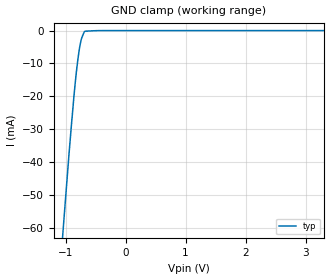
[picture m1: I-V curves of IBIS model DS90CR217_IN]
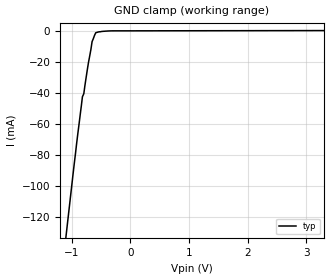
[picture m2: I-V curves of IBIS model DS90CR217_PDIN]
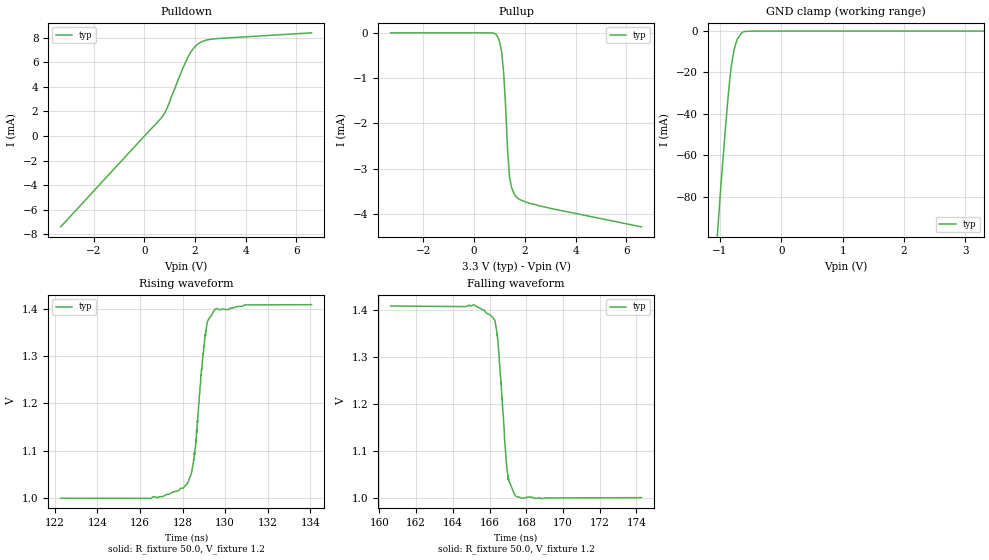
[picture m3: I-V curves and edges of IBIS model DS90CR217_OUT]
|   National Semiconductor Corporation
|   Interface Products Group
|   IBIS Model of DS90CR217MTD
|   High Speed Link Transmitter
|   48L TSSOP
[IBIS Ver]   2.1
[Comment char]  |_char
[File name]   90cr217.ibs
[File Rev]   1.3
[Date]   7/27/00
[Source]   File originated at National Semiconductor Corporation.
   Interface Group/Analog Division. All data based on
   Empirical Measurements(Bench).
[Notes]   File created by DT.
   Revision 1.0: The original model.
   Revision 1.1: Modified driver output pulldown
   and pullup to ensure no double
   counting of clamp current.
   Revision 1.2: Corrected ground and power clamp data.
   Revision 1.3: Changed Vdiff in pin mapping for LVDS
   Outputs from .1 to 0
   Changed Vref in V/T data from 0 to 1.2
[Disclaimer]
(C) Copyright National Semiconductor Corporation 2000
   All rights reserved
   National Semiconductor Corporation hereby grants
the user of this IBIS model a non-exclusive, nontransferable
license to use this IBIS model under the following terms.
Before using this IBIS model, the user should read this
license.  If the user does not accept these terms, the
IBIS model should be returned to National within 30 days.
   The user is granted this license only to use the
IBIS model and is not granted rights to sell, load, rent,
lease or license the IBIS model in whole or in part, or in
modified form to anyone other than user. User may modify
the IBIS model to suit its specific applications but rights
to derivative works and such modifications shall belong to
National.
   This IBIS model is provided on an "AS IS" basis and
National makes absolutely no warranty with respect to the
information contained herein. NATIONAL DISCLAIMS AND CUSTOMER
WAIVES ALL WARRANTIES, EXPRESS OR IMPLIED, INCLUDING
WARRANTIES OF MERCHANTABILITY OR FITNESS FOR A PARTICULAR
PURPOSE. The entire risk as to quality and performance is
with the Customer. ACCORDINGLY, IN NO EVENT SHALL THE
COMPANY BE LIABLE FOR ANY DAMAGES, WHETHER IN CONTRACT OR
TORT,INCLUDING ANY LOST PROFITS OR OTHER INCIDENTAL,
CONSEQUENTIAL, EXEMPLARY, OR PUNITIVE DAMAGES ARISING OUT
OF THE USE OR APPLICATION OF THE IBIS model provided in
this package. Further, National reserves the right to make
changes without notice to any product herein to improve
reliability, function, or design. National does not convey
any license under patent rights or any other intellectual
property rights, including those of third parties.
   National is not obligated to provide maintenance or support
for the licensed IBIS model.
Contact National at ATTN:INTERFACE APPLICATIONS/IBIS MODELS.
2900 Semiconductor Drive, M/S A2595, Santa Clara, CA 95052-8090
[Copyright]   Copyright 2000, National Semiconductor, All Rights Reserved
[Component]   DS90CR217MTD
[Manufacturer]  National Semiconductor Corp
[Package]
|   typ   min   max
R_pkg   97.97m   NA   NA
L_pkg   3.000nH   NA   NA
C_pkg   0.2108pF   NA   NA
[Pin]   signal_name   model_name   R_pin   L_pin   C_pin
1   TxIN4   DS90CR217_IN   68.8m   2.270n   0.3587p
2   Vcc   POWER   65.4m   2.200n   0.3414p
3   TxIN5   DS90CR217_IN   133.7m   3.880n   0.3183p
4   TxIN6   DS90CR217_IN   121.7m   3.590n   0.2610p
5   GND   GND   120.6m   3.510n   0.2205p
6   TxIN7   DS90CR217_IN   117.6m   3.460n   0.1689p
7   TxIN8   DS90CR217_IN   104.9m   3.170n   0.1594p
8   Vcc   POWER   97.8m   2.970n   0.1515p
9   TxIN9   DS90CR217_IN   92.6m   2.860n   0.1459p
10   TxIN10   DS90CR217_IN   92.6m   2.840n   0.1459p
11   GND   GND   94.0m   2.800n   0.1568p
12   TxIN11   DS90CR217_IN   81.7m   2.640n   0.1311p
13   TxIN12   DS90CR217_IN   73.9m   2.660n   0.1116p
14   Vcc   POWER   89.6m   2.720n   0.1343p
15   TxIN13   DS90CR217_IN   87.2m   2.860n   0.1384p
16   TxIN14   DS90CR217_IN   92.6m   2.880n   0.1458p
17   GND   GND   98.8m   3.040n   0.1563p
18   TxIN15   DS90CR217_IN   102.9m   3.160n   0.1572p
19   TxIN16   DS90CR217_IN   111.4m   3.210n   0.1639p
20   TxIN17   DS90CR217_IN   113.5m   3.340n   0.2126p
21   Vcc   POWER   121.8m   3.590n   0.2606p
22   TxIN18   DS90CR217_IN   133.8m   3.880n   0.3183p
23   TxIN19   DS90CR217_IN   65.5m   2.200n   0.3414p
24   GND   GND   68.8m   2.270n   0.3587p
25   TxIN20   DS90CR217_IN   68.8m   2.270n   0.3587p
26   TxCLKIN   DS90CR217_IN   65.5m   2.200n   0.3414p
27   PWRDWN*   DS90CR217_PDIN   133.8m   3.880n   0.3183p
28   PLLGND   GND   121.8m   3.590n   0.2606p
29   PLLVCC   POWER   113.5m   3.340n   0.2126p
30   PLLGND   GND   111.4m   3.210n   0.1639p
31   LVDSGND   GND   102.9m   3.160n   0.1572p
32   TxCLKOUT+   DS90CR217_OUT   98.8m   3.040n   0.1563p
33   TxCLKOUT-   DS90CR217_OUT   92.6m   2.880n   0.1458p
34   TxOUT2+   DS90CR217_OUT   87.2m   2.860n   0.1384p
35   TxOUT2-   DS90CR217_OUT   89.6m   2.720n   0.1343p
36   LVDSGND   GND   73.9m   2.660n   0.1116p
37   LVDSVCC   POWER   81.7m   2.640n   0.1311p
38   TxOUT1+   DS90CR217_OUT   94.0m   2.800n   0.1568p
39   TxOUT1-   DS90CR217_OUT   92.6m   2.840n   0.1459p
40   TxOUT0+   DS90CR217_OUT   92.6m   2.860n   0.1459p
41   TxOUT0-   DS90CR217_OUT   97.8m   2.970n   0.1515p
42   LVDSGND   GND   104.9m   3.170n   0.1594p
43   N/C   NC   117.6m   3.460n   0.1689p
44   TxIN0   DS90CR217_IN   120.6m   3.510n   0.2205p
45   TxIN1   DS90CR217_IN   121.7m   3.590n   0.2610p
46   GND   GND   133.7m   3.880n   0.3183p
47   TxIN2   DS90CR217_IN   65.4m   2.200n   0.3414p
48   TxIN3   DS90CR217_IN   68.8m   2.270n   0.3587p
[Diff_pin]   inv_pin   vdiff   tdelay_typ   tdelay_min   tdelay_max
| The '+' pin is Diff_pin and the '-' pin is the inv_pin
32   33   0.0   0   0   0
34   35   0.0   0   0   0
38   39   0.0   0   0   0
40   41   0.0   0   0   0
| Models and submodels in the file (3): DS90CR217_IN (Input), DS90CR217_PDIN (Input), DS90CR217_OUT (3-state)
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|   Driver Input  MODEL
[Model]   DS90CR217_IN
Model_type   Input
|Signals   TxIN0 ~ TxIN20
Vinh = 2.0
Vinl = 0.8
|   typ   min   max
C_comp   5.747pF   NA   NA
|   typ   min   max
[Temperature Range]   25.0   NA   NA
[Voltage range]   3.3V   3.0V   3.6V
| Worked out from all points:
|   GND clamp passes 1 mA (typ) near -0.70 V on its own axis
[Power_clamp]
| Note that the[POWER_clamp]voltage table is referenced to Vcc
| and is calculated using Vtable=Vcc - Vmeasured.
|Voltage   I(typ)   I(min)   I(max)
-3V       0A         NA         NA
3V        0A         NA         NA
[GND_clamp]
|Voltage   I(typ)   I(min)   I(max)
-3.3V     -594.1mA   NA         NA
-1.001V   -51.39mA   NA         NA
-941.2mV  -37.29mA   NA         NA
-899.9mV  -28.27mA   NA         NA
-859.6mV  -19.87mA   NA         NA
-818.3mV  -12.37mA   NA         NA
-776.9mV  -6.424mA   NA         NA
-756.3mV  -4.202mA   NA         NA
-736.1mV  -2.573mA   NA         NA
-717mV    -1.615mA   NA         NA
-675.2mV  -194.8uA   NA         NA
3.3V      524nA      NA         NA
|   Driver PWRDWN* Input  MODEL
[Model]   DS90CR217_PDIN
Model_type   Input
|Signals   PWRDWN*
Vinh = 2.0
Vinl = 0.8
|   typ   min   max
C_comp   5.679pF   NA   NA
|   typ   min   max
[Temperature Range]   25.0   NA   NA
[Voltage range]   3.3V   3.0V   3.6V
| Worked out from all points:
|   GND clamp passes 1 mA (typ) near -0.57 V on its own axis
[Power_clamp]
| Note that the[POWER_clamp]voltage table is referenced to Vcc
| and is calculated using Vtable=Vcc - Vmeasured.
|Voltage   I(typ)   I(min)   I(max)
-3V       0A         NA         NA
3V        0A         NA         NA
[GND_clamp]
|Voltage   I(typ)   I(min)   I(max)
-3.3V     -863.2mA   NA         NA
-999.7mV  -98.78mA   NA         NA
-918.6mV  -72.42mA   NA         NA
-819.7mV  -42.41mA   NA         NA
-796.1mV  -40.44mA   NA         NA
-776.9mV  -35.09mA   NA         NA
-735.6mV  -24.85mA   NA         NA
-674.7mV  -11.91mA   NA         NA
-655mV    -6.957mA   NA         NA
-592.5mV  -1.248mA   NA         NA
-306.8mV  -9.428uA   NA         NA
3.3V      172.6uA    NA         NA
|   Driver Output  MODEL
[Model]   DS90CR217_OUT
Model_type   3-state
| Signals   TxOUT0 ~ TxOUT2; TxCLKOUT
Vmeas = 1.2V   |This is 0.0v differential on output
Cref = 5pF   |Timing specification test load capacitance value
Rref = 50   |Note: 100 Ohm between the two driver outputs
Vref = 1.2   |Timing specification test load voltage; GND
| variable   typ   min   max
C_comp   6.236pF   NA   NA
|   typ   min   max
[Temperature Range]   25.0   NA   NA
[Voltage range]   3.3V   3.0V   3.6V
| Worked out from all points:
|   slope of the pulldown table from 0 to 0.495 V, typ, clamps not added: 459 ohm
|   GND clamp passes 1 mA (typ) near -0.65 V on its own axis
|   rising waveform, R_fixture 50.0, V_fixture 1.2: 20-80 % time 486ps typ, NA min, NA max; typ from 1 V to 1.41 V
|   falling waveform, R_fixture 50.0, V_fixture 1.2: 20-80 % time 438ps typ, NA min, NA max; typ from 1.41 V to 1 V
[Pulldown]
| Voltage   I(typ)   I(min)   I(max)
-3.3V     -7.392mA   NA         NA
667.8mV   1.466mA    NA         NA
748mV     1.688mA    NA         NA
907.8mV   2.312mA    NA         NA
1.372V    4.782mA    NA         NA
1.681V    6.257mA    NA         NA
1.909V    7.054mA    NA         NA
2.136V    7.516mA    NA         NA
2.442V    7.802mA    NA         NA
2.749V    7.903mA    NA         NA
6.6V      8.398mA    NA         NA
[Pullup]
| Note that the[Pullup]voltage table is referenced to Vcc
| and is calculated using Vtable=Vcc - Vmeasured.
|Voltage   I(typ)   I(min)   I(max)
-3.3V     -524nA     NA         NA
854.5mV   -29.33uA   NA         NA
1.009V    -203.2uA   NA         NA
1.087V    -429.5uA   NA         NA
1.164V    -876.3uA   NA         NA
1.242V    -1.62mA    NA         NA
1.32V     -2.587mA   NA         NA
1.396V    -3.187mA   NA         NA
1.474V    -3.411mA   NA         NA
1.629V    -3.606mA   NA         NA
2.559V    -3.822mA   NA         NA
6.6V      -4.289mA   NA         NA
[GND_clamp]
| Outputs in Tri-state.
| Voltage   I(typ)   I(min)   I(max)
-3.3V     -1.034A    NA         NA
-1.001V   -81.02mA   NA         NA
-983mV    -73.48mA   NA         NA
-921.5mV  -50.22mA   NA         NA
-900.9mV  -42.95mA   NA         NA
-859.6mV  -29.11mA   NA         NA
-819.2mV  -17.54mA   NA         NA
-767.2mV  -8.785mA   NA         NA
-719.4mV  -3.945mA   NA         NA
-634.3mV  -657.5uA   NA         NA
-347.7mV  -11.87uA   NA         NA
3.3V      524nA      NA         NA
[POWER_clamp]
| Note that the[POWER_clamp]voltage table is referenced to Vcc
| and is calculated using Vtable=Vcc - Vmeasured.
| Outputs in Tri-state.
|Voltage   I(typ)   I(min)   I(max)
-3V       0A         NA         NA
3V        0A         NA         NA
[Ramp]
| Note: Ramp rate measured on single-ended Driver Output.
|   typ   min   max
dV/dt_r   204.0m/446.03p   NA   NA
dV/dt_f   205.5m/372.29p   NA   NA
R_load = 100Ohm | Note: This 100 Ohm is across the two driver output
[Rising Waveform]
R_fixture = 50.0
V_fixture = 1.2
|C_fixture = 8.0pF
|Time   V(typ)   V(min)  V(max)
122.3ns   999.6mV    NA         NA
126.5ns   998.6mV    NA         NA
128ns     1.021V     NA         NA
128.4ns   1.048V     NA         NA
128.5ns   1.081V     NA         NA
128.6ns   1.118V     NA         NA
128.9ns   1.259V     NA         NA
129.1ns   1.347V     NA         NA
129.5ns   1.399V     NA         NA
134.1ns   1.409V     NA         NA
[Falling Waveform]
R_fixture = 50.0
V_fixture = 1.2
|C_fixture = 8.0pF
|Time   V(typ)   V(min)  V(max)
160.6ns   1.41V      NA         NA
165.1ns   1.412V     NA         NA
166.3ns   1.379V     NA         NA
166.4ns   1.349V     NA         NA
166.5ns   1.314V     NA         NA
166.8ns   1.122V     NA         NA
166.9ns   1.059V     NA         NA
167ns     1.039V     NA         NA
167.4ns   1.005V     NA         NA
174.3ns   1.001V     NA         NA
